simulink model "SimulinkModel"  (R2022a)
settings: Solver=FixedStepAuto  StartTime=0.0  StopTime=Inf  RelTol=1e-3  EnableMultiTasking=on
libraries: c2837xDlib x1

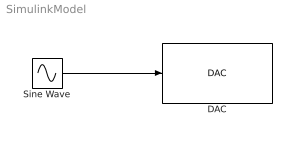
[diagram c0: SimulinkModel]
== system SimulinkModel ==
  DAC : c2837xDlib/DAC  channel=A  saturate=on
  Sine Wave : Sin  SineType=Sample based  Amplitude=2047.5  Bias=2047.5  Samples=100  SampleTime=.01
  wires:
  Sine Wave/1 -> DAC/1
